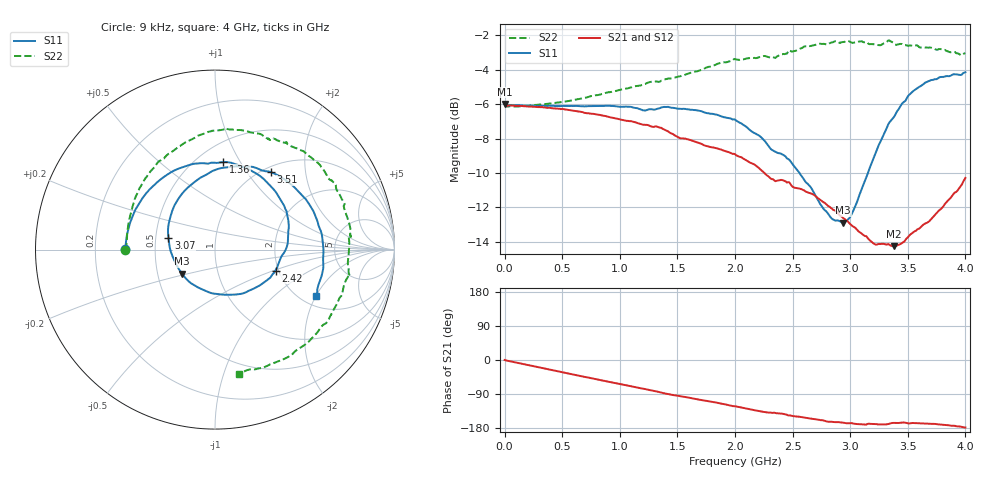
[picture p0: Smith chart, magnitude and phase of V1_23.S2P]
! ZVRE, 3.40
! symbol freq-unit parameter-type data-format keyword impedance-ohm
#  HZ  S  RI  R  50
! freq  reS11  imS11  reS21  imS21  reS12  imS12  reS22  imS22
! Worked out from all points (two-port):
!   401 points, 9 kHz to 4 GHz, reference 50 ohm
!   highest |S21| = -5.98 dB at 9 kHz (marker M1); lowest = -14.3 dB at 3.38 GHz (marker M2)
!   |S21| within 3 dB of the highest: start of sweep to 2.014 GHz
!   lowest |S11| = -12.9 dB at 2.94 GHz (marker M3), VSWR 1.59, Z = 33.5 - j9.52 ohm
!   |S11| at or under -10 dB: 2.56 GHz to 3.154 GHz (593.5 MHz wide, 20.8 % of centre)
!   |S22| runs from -6.1 to -2.3 dB; largest |S21 - S12| = 0.011
!   S11 on the Smith chart (normalised r, x): 9 kHz: 0.33, +0.00; 1.36 GHz: 0.66, +0.85; 2.42 GHz: 1.93, -0.52; 3.07 GHz: 0.58, +0.08; 3.51 GHz: 1.09, +1.31; 4 GHz: 2.39, -2.01
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9000  -0.5003 0.0014  0.5022 0.000581  0.503 -0.00207  -0.5013 -0.000431
3.400082e8  -0.4551 0.1954  0.4548 -0.1841  0.4593 -0.1819  -0.4848 0.1267
6.700075e8  -0.3454 0.3534  0.3472 -0.325  0.3525 -0.3225  -0.4552 0.2537
1.040007e9  -0.1486 0.4697  0.1852 -0.4098  0.1898 -0.4111  -0.3878 0.3978
1.340006e9  0.0327 0.4859  0.0422 -0.427  0.0451 -0.4296  -0.2846 0.5074
1.360006e9  0.0449 0.4882  0.0302 -0.4267  0.0338 -0.4271  -0.2786 0.516
1.660005e9  0.2442 0.415  -0.0865 -0.3796  -0.0832 -0.3813  -0.1496 0.6057
2.000004e9  0.3995 0.211  -0.1913 -0.3034  -0.188 -0.3059  0.064 0.6752
2.210004e9  0.4047 0.0329  -0.2301 -0.2316  -0.2282 -0.2351  0.2204 0.6502
2.420004e9  0.3372 -0.1169  -0.238 -0.1845  -0.2377 -0.1866  0.3366 0.6153
2.670003e9  0.1368 -0.2478  -0.2493 -0.1155  -0.2491 -0.122  0.5373 0.5119
2.810003e9  -0.0338 -0.2378  -0.2422 -0.0745  -0.243 -0.0851  0.6397 0.3889
2.940002e9  -0.1826 -0.1348  -0.2263 -0.0589  -0.2298 -0.058  0.6991 0.2966
3.070002e9  -0.2591 0.0645  -0.2107 -0.0397  -0.2146 -0.0403  0.7465 0.1481
3.190002e9  -0.2167 0.2624  -0.1952 -0.0391  -0.1978 -0.0412  0.7483 0.0351
3.340001e9  -0.000705 0.4434  -0.1917 -0.0398  -0.195 -0.0401  0.7538 -0.1446
3.380001e9  0.0555 0.4566  -0.188 -0.0469  -0.1897 -0.0474  0.7326 -0.165
3.510001e9  0.3123 0.4317  -0.2026 -0.0443  -0.2061 -0.0517  0.6488 -0.3583
3.640001e9  0.4944 0.2924  -0.2193 -0.0477  -0.2227 -0.0479  0.5662 -0.4663
3.760001e9  0.5833 0.1179  -0.2398 -0.0436  -0.2427 -0.0437  0.442 -0.5706
3.89e9  0.6039 -0.0933  -0.2712 -0.0307  -0.2745 -0.0261  0.2811 -0.652
4e9  0.5639 -0.2588  -0.3058 -0.00989  -0.3041 -0.00379  0.1349 -0.6925
